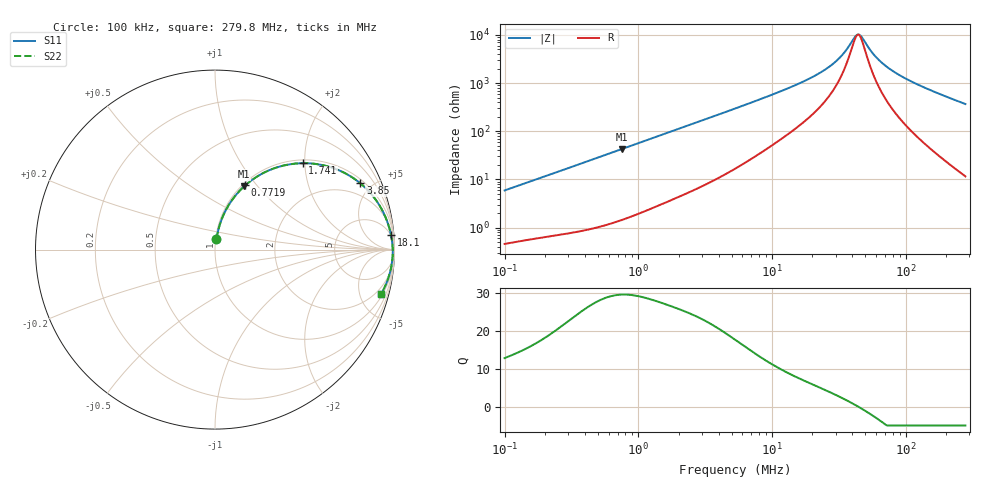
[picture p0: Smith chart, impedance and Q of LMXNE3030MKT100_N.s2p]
! LMXNE3030MKT100_N  S-PARAMETER MODEL  ( General Type )
! Model Generated by TAIYO YUDEN Corporation (https://www.yuden.co.jp/en/)
! Version 1.0
! TAIYO YUDEN Control No. 191023NI43SB-FBB
! Copyright(c) 2019 TAIYO YUDEN CO.,LTD. All Rights Reserved.
! Product Description (link to TY-COMPAS)
! https://ds.yuden.co.jp/TYCOMPAS/or/detail?pn=LMXNE3030MKT100MN&u=M
! Products Name : Inductors
! Characteristics :
!  Inductance : 10 uH , SRF(min) : 32 MHz , DC Resistance(max) : 0.324 Ohm
!  Rated Current : Saturation :730 mA , Temp Rise : 720 mA (40 degC)
!  Case Size : 3.0 x 3.0 / 0.118 x 0.118 [mm/inch] , Thickness : 1.2 / 0.047 [mm/inch]
!  (Conditions: Temperature = 25 degC , DC Bias Current/Voltage = 0A / 0V)
! External Node Assignments :
!  1  o---GGG---o  2
! GND o---------o GND
! Frequency Range : 0.1MHz  -  279.750408MHz  [ 402 STEP ]
# MHz S RI R 50
! Freq[MHz].  S11 Real  S11 Imag  S21 Real  S21 Imag  S12 Real  S12 Imag  S22 Real  S22 Imag
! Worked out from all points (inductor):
!   401 points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, 100 kHz to 279.8 MHz, reference 50 ohm
!   read as one part in series: L = 9.29 uH near 104 kHz
!   highest Q = 29.7 at 756.7 kHz (marker M1), where L = 9.01 uH
!   self-resonance near 43.33 MHz
!   S11 on the Smith chart (normalised r, x): 100 kHz: 1.01, +0.12; 771.9 kHz: 1.03, +0.87; 1.741 MHz: 1.07, +1.95; 3.85 MHz: 1.20, +4.28; 18.1 MHz: 4, +23; 279.8 MHz: 1.23, -7.33
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0.1  0.00796 0.0581  0.992 -0.0581  0.992 -0.0581  0.00796 0.0581
0.377863  0.0518 0.2027  0.9482 -0.2027  0.9482 -0.2027  0.0518 0.2027
0.756705  0.1635 0.3533  0.8365 -0.3533  0.8365 -0.3533  0.1635 0.3533
0.771869  0.1687 0.358  0.8313 -0.358  0.8313 -0.358  0.1687 0.358
1.427803  0.3952 0.4712  0.6048 -0.4712  0.6048 -0.4712  0.3952 0.4712
1.741155  0.488 0.4815  0.512 -0.4815  0.512 -0.4815  0.488 0.4815
2.488526  0.6524 0.4563  0.3476 -0.4563  0.3476 -0.4563  0.6524 0.4563
3.850477  0.8099 0.3693  0.1901 -0.3693  0.1901 -0.3693  0.8099 0.3693
5.289144  0.8839 0.2934  0.1161 -0.2934  0.1161 -0.2934  0.8839 0.2934
10.80425  0.9612 0.1514  0.0388 -0.1514  0.0388 -0.1514  0.9612 0.1514
18.09818  0.9802 0.0829  0.0198 -0.0829  0.0198 -0.0829  0.9802 0.0829
19.9857  0.9823 0.0722  0.0177 -0.0722  0.0177 -0.0722  0.9823 0.0722
25.35844  0.9862 0.0485  0.0138 -0.0485  0.0138 -0.0485  0.9862 0.0485
30.31621  0.9881 0.0323  0.0119 -0.0323  0.0119 -0.0323  0.9881 0.0323
34.8332  0.9892 0.0201  0.0108 -0.0201  0.0108 -0.0201  0.9892 0.0201
41.64336  0.9901 0.00485  0.00988 -0.00485  0.00988 -0.00485  0.9901 0.00485
44.19738  0.9903 -0.00022  0.00971 0.00022  0.00971 0.00022  0.9903 -0.00022
46.90804  0.9904 -0.00531  0.0096 0.00531  0.0096 0.00531  0.9904 -0.00531
60.711  0.9901 -0.0279  0.00989 0.0279  0.00989 0.0279  0.9901 -0.0279
75.51853  0.9888 -0.0485  0.0112 0.0485  0.0112 0.0485  0.9888 -0.0485
126.5009  0.9797 -0.1076  0.0203 0.1076  0.0203 0.1076  0.9797 -0.1076
279.7504  0.9241 -0.2496  0.0759 0.2496  0.0759 0.2496  0.9241 -0.2496
